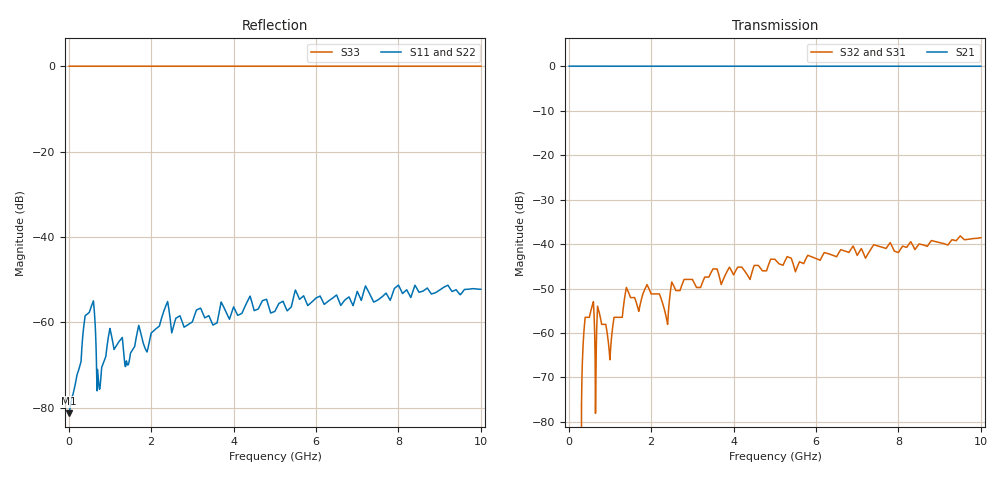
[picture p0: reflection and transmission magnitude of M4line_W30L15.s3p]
! Created Fri Sep 09 14:31:10 2011
# ghz S ma R 50
! 3 Port Network Data from SP1.SP block
! freq  magS11  angS11  magS12  angS12  magS13  angS13
!  magS21  angS21
!  magS22  angS22  magS23  angS23
!  magS31  angS31  magS32  angS32
!  magS33  angS33
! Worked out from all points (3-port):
!   1000 points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, 10 MHz to 10 GHz, reference 50 ohm
!   strongest paths, dB at 10 MHz, 2.51 GHz, 5.01 GHz, 7.51 GHz, 10 GHz:
!     S21: 0.0, 0.0, 0.0, 0.0, 0.0
!     S32: -, -48.7, -43.5, -40.5, -38.6
!     S31: -, -48.7, -43.5, -40.5, -38.6
!   lowest |S11| = -81.3 dB at 10 MHz (marker M1), VSWR 1.00, Z = 50 + j0.00113 ohm
!   |S11| at or under -10 dB: start of sweep to end of sweep
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0.01  8.608e-05 7.5  0.9999 -0.0  0 0.0
      0.9999 -0.0  8.608e-05 7.5  0 0.0
      0 0.0  0 0.0  1 0.0
0.26  0.0002968 70.6  0.9999 -0.0  0 0.0
      0.9999 -0.0  0.0002968 70.6  0 0.0
      0 0.0  0 0.0  1 0.0
0.39  0.001112 84.4  0.9999 0.0  0.00135 -89.9
      0.9999 0.0  0.001112 84.4  0.00135 -89.9
      0.00135 -89.9  0.00135 -89.9  1 0.2
0.56  0.001592 85.3  0.9999 0.0  0.00195 -89.8
      0.9999 0.0  0.001592 85.3  0.00195 -89.8
      0.00195 -89.8  0.00195 -89.8  1 0.2
0.73  0.0001866 -30.7  0.9998 -0.1  0.001775 89.8
      0.9998 -0.1  0.0001866 -30.7  0.001775 89.8
      0.001775 89.8  0.001775 89.8  1 -0.2
1  0.0008475 75.1  0.9998 -0.1  0.0005 90.0
   0.9998 -0.1  0.0008475 75.1  0.0005 90.0
   0.0005 90.0  0.0005 90.0  1 -0.1
1.42  0.0003233 -15.5  0.9997 -0.2  0.0031 89.7
      0.9997 -0.2  0.0003233 -15.5  0.0031 89.7
      0.0031 89.7  0.0031 89.7  1 -0.4
2.37  0.001622 70.1  0.9994 -0.2  0.001475 89.9
      0.9994 -0.2  0.001622 70.1  0.001475 89.9
      0.001475 89.9  0.001475 89.9  1 -0.2
5.01  0.001372 38.1  0.9989 -0.4  0.006675 89.4
      0.9989 -0.4  0.001372 38.1  0.006675 89.4
      0.006675 89.4  0.006675 89.4  1 -0.8
10  0.002439 38.9  0.9979 -0.8  0.0118 88.5
    0.9979 -0.8  0.002439 38.9  0.0118 88.5
    0.0118 88.5  0.0118 88.5  0.9997 -1.4
